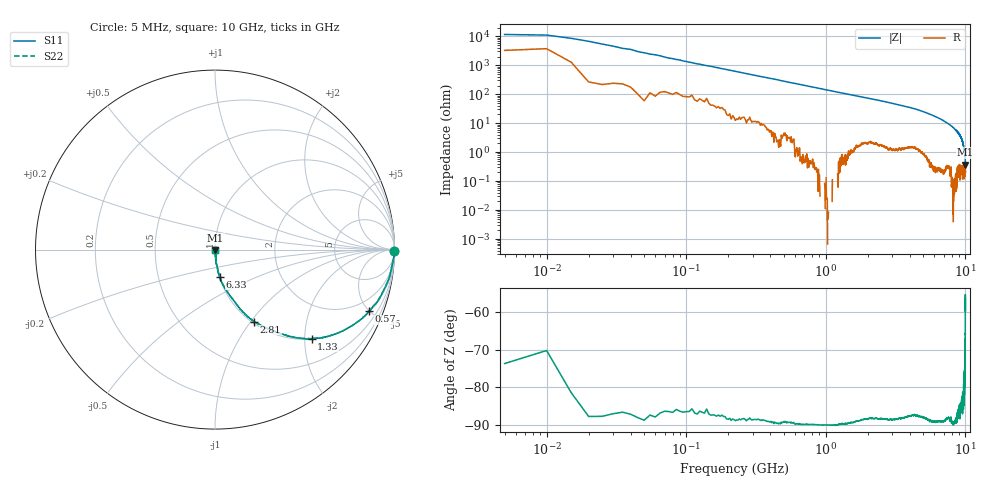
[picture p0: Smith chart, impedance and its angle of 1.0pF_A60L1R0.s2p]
! Amotech Co.,Ltd.
! http://www.amotech.co.kr/
! Part Number: A60L1R0
! These Parameters are Measured in Series Mode Connection
! Operation Temp=25[degC], DC Bias Voltage=0[V]
! Freq. Start=5[MHz] Stop=10[GHz], 2000[Steps]
! Date: Monday, July 14, 2020, 09:45:01
# GHZ S RI R 50.000000
!Freq.(Hz) S11(Real) S11(Imag) S21(Real) S21(Imag) S12(Real) S12(Imag) S22(Real) S22(Imag)
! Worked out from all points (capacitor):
!   2000 points, 5 MHz to 10 GHz, reference 50 ohm
!   read as one part in series: C = 1.18 pF near 55 MHz
!   lowest |Z| = 374 mohm at 9.995 GHz (marker M1)
!   S11 on the Smith chart (normalised r, x): 5 MHz: open; 570 MHz: 1.05, -4.97; 1.33 GHz: 1.01, -2.16; 2.81 GHz: 1.03, -1.04; 6.33 GHz: 1.01, -0.31; 10 GHz: 1.00, -0.01
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0.005  0.9975 -0.00826  0.0025 0.00826  0.0025 0.00826  0.9975 -0.00826
0.085  0.9916 -0.0621  0.00843 0.0621  0.00843 0.0621  0.9916 -0.0621
0.12  0.9877 -0.0876  0.0123 0.0876  0.0123 0.0876  0.9877 -0.0876
0.165  0.9811 -0.1171  0.0189 0.1171  0.0189 0.1171  0.9811 -0.1171
0.325  0.9432 -0.2185  0.0568 0.2185  0.0568 0.2185  0.9432 -0.2185
0.57  0.8582 -0.3437  0.1418 0.3437  0.1418 0.3437  0.8582 -0.3437
0.925  0.705 -0.4563  0.295 0.4563  0.295 0.4563  0.705 -0.4563
1.33  0.5386 -0.4958  0.4614 0.4958  0.4614 0.4958  0.5386 -0.4958
1.675  0.4306 -0.486  0.5694 0.486  0.5694 0.486  0.4306 -0.486
2.81  0.2187 -0.4014  0.7813 0.4014  0.7813 0.4014  0.2187 -0.4014
3.34  0.1633 -0.3544  0.8367 0.3544  0.8367 0.3544  0.1633 -0.3544
5.005  0.0655 -0.2305  0.9345 0.2305  0.9345 0.2305  0.0655 -0.2305
6.33  0.0261 -0.1508  0.9739 0.1508  0.9739 0.1508  0.0261 -0.1508
6.67  0.0208 -0.1343  0.9792 0.1343  0.9792 0.1343  0.0208 -0.1343
8.335  0.00451 -0.0633  0.9955 0.0633  0.9955 0.0633  0.00451 -0.0633
8.945  0.00435 -0.0446  0.9957 0.0446  0.9957 0.0446  0.00435 -0.0446
9.49  0.004 -0.0248  0.996 0.0248  0.996 0.0248  0.004 -0.0248
9.665  0.00244 -0.0171  0.9976 0.0171  0.9976 0.0171  0.00244 -0.0171
9.825  0.00269 -0.0115  0.9973 0.0115  0.9973 0.0115  0.00269 -0.0115
9.92  0.00264 -0.00698  0.9974 0.00698  0.9974 0.00698  0.00264 -0.00698
9.995  0.00189 -0.00322  0.9981 0.00322  0.9981 0.00322  0.00189 -0.00322
10  0.00224 -0.00333  0.9978 0.00333  0.9978 0.00333  0.00224 -0.00333
